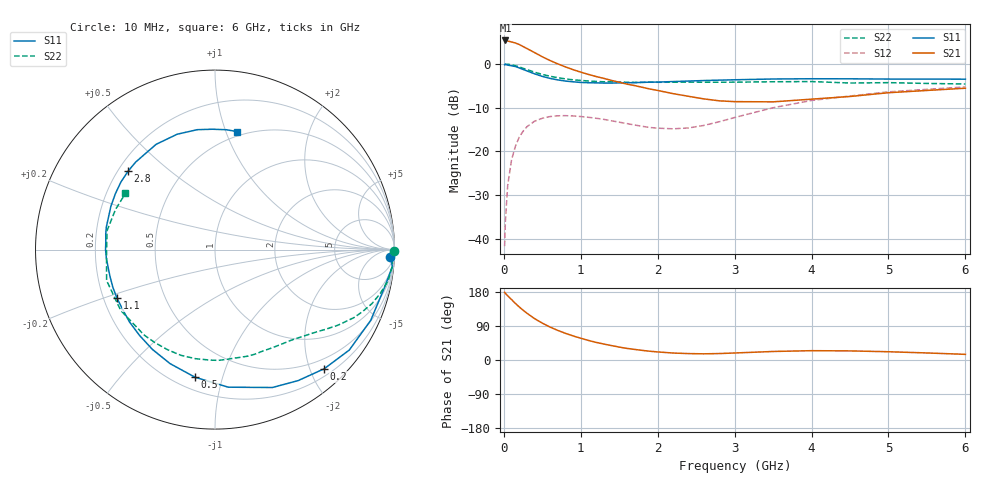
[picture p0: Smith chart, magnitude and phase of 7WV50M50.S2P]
! Infineon Technologies  Discrete & RF Semiconductors
! BFS17W
! Si NPN RF Bipolar Junction Transistor in SOT323
! VCE = 0.5 V  IC = 0.5 mA
! Common Emitter S-Parameters:  August  1999
# GHz  S  MA  R  50
!  f  S11  S21  S12  S22
! GHz  MAG  ANG  MAG  ANG  MAG  ANG  MAG  ANG
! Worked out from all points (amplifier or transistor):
!   36 points, 10 MHz to 6 GHz, reference 50 ohm
!   highest |S21| = 5.4 dB at 20 MHz (marker M1)
!   |S21| within 3 dB of that: start of sweep to 422.8 MHz
!   unconditionally stable (mu >= 1): 994.7 MHz to end of sweep
!   at 250 MHz: K = 0.29, MSG = 9.7 dB, |S12| = -15.4 dB
!   at 1.4 GHz: K = 1.33, MAG = 1.2 dB, |S12| = -13.0 dB
!   at 6 GHz: K = 1.15, MAG = -2.5 dB, |S12| = -5.3 dB
!   S11 on the Smith chart (normalised r, x): 10 MHz: 22, -36; 200 MHz: 0.32, -2.23; 500 MHz: 0.28, -0.82; 1.1 GHz: 0.26, -0.22; 2.8 GHz: 0.24, +0.36; 6 GHz: 0.46, +1.09
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0.01  0.9758 -2.3  1.829 178.8  0.0082 87.0  1 -0.5
0.02  0.9929 -5.4  1.856 175.9  0.0156 90.4  0.9854 -2.0
0.05  0.9683 -12.4  1.828 169.5  0.0406 81.6  0.9929 -5.2
0.1  0.953 -24.4  1.786 159.6  0.0797 74.5  0.9797 -10.2
0.15  0.9343 -36.8  1.735 149.3  0.1139 66.3  0.9524 -14.9
0.2  0.9005 -47.5  1.668 140.0  0.1449 60.2  0.9248 -19.0
0.25  0.8644 -57.6  1.581 131.5  0.1694 53.5  0.8915 -22.8
0.3  0.8323 -67.4  1.501 123.5  0.1911 48.4  0.8627 -26.0
0.4  0.7701 -84.5  1.347 109.1  0.221 38.7  0.8041 -31.6
0.5  0.72 -98.8  1.208 97.3  0.2387 31.4  0.7582 -35.9
0.6  0.6829 -111.5  1.094 87.0  0.2498 25.7  0.7226 -39.7
0.8  0.6367 -131.4  0.925 70.4  0.2557 17.1  0.674 -47.0
1.1  0.6092 -153.8  0.758 51.6  0.2449 9.3  0.6378 -57.5
1.6  0.6098 -180.0  0.587 30.6  0.2075 6.9  0.6167 -76.5
2.2  0.6282 157.4  0.457 18.4  0.1808 21.5  0.6174 -99.9
2.8  0.6521 138.0  0.378 17.0  0.2178 39.2  0.617 -122.9
3.5  0.6721 119.2  0.368 22.5  0.3152 43.0  0.625 -147.2
4  0.6765 108.1  0.395 24.6  0.3815 38.9  0.628 -164.1
4.5  0.6754 98.4  0.424 24.0  0.4295 33.6  0.6044 -178.8
5  0.6708 91.2  0.468 21.8  0.4788 28.5  0.6105 170.1
5.5  0.6708 84.6  0.497 18.6  0.5122 23.4  0.5977 158.0
6  0.6688 79.4  0.527 14.9  0.5454 18.4  0.5891 147.9
